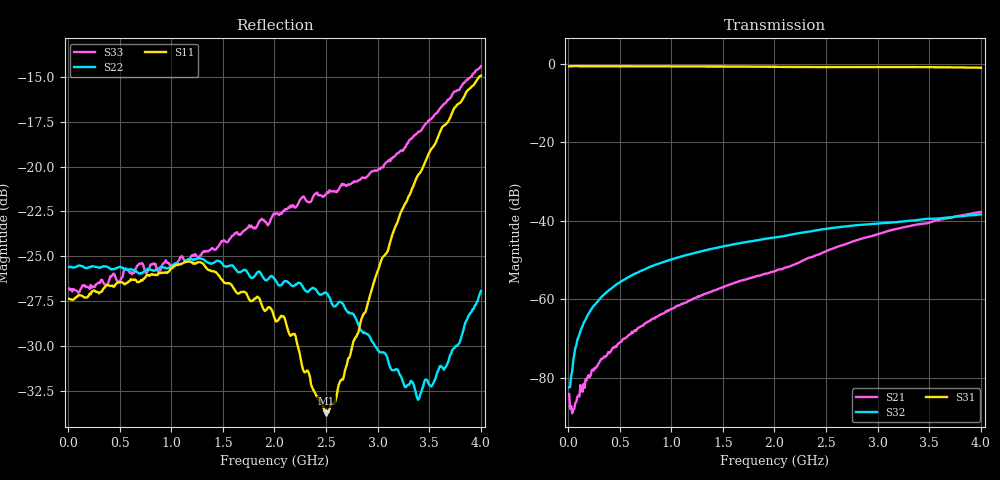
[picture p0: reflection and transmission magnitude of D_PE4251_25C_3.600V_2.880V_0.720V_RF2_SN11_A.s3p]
! Device ID: PE4251_SoldCshunt_081809
! Dir: c:\Test Bench Repositories\Bench_Software_CVI_Version_8\trunk\PSC 4Port_VNA Bench\datalog\4250\TEST\PE4251_SoldCshunt_081809\25C\3p600000\RF2
! Serial: 11
! Insertion: A
! Temp: 25C
! VDD: 3.600
! Control_Hi: 80.000
! Control_Lo: 20.000
! Logic State: RF2
! Port 1: RFC
! Port 2: RF1
! Port 3: RF2
! V1 = 0.72
! V2 = 0.72
! V3 = 0.72
! IDD: 4.934160e-05
! FILE NAME
! DATE 08/18/09  20:13
! CORRECTED  DATA
#  Hz  S  RI  R  50.00
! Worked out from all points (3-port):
!   401 points, 10 MHz to 4 GHz, reference 50 ohm
!   strongest paths, dB at 10 MHz, 1.008 GHz, 2.005 GHz, 3.002 GHz, 4 GHz:
!     S31: -0.6, -0.6, -0.7, -0.8, -0.9
!     S32: -82.5, -49.8, -44.2, -40.7, -38.3
!     S21: -84.2, -62.4, -52.8, -43.4, -37.7
!   lowest |S11| = -33.7 dB at 2.504 GHz (marker M1), VSWR 1.04, Z = 50.5 - j2 ohm
!   |S11| at or under -10 dB: start of sweep to end of sweep
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1e7  0.0428 -0.00063  9.73e-05 6.83e-05  0.9368 -0.00251
     6.12e-05 -8.49e-06  0.0525 -0.000729  3.26e-05 1.67e-05
     0.9381 -0.00458  5.86e-06 -7.49e-05  0.0457 0.000517
8.98e7  0.0435 0.00135  1.78e-05 -5.36e-05  0.9389 -0.0323
        2.09e-05 -5.28e-05  0.0528 -0.00117  3.32e-05 0.000282
        0.939 -0.0326  4.61e-05 0.000301  0.0449 -0.000647
1.696e8  0.0432 0.0021  2.64e-06 -8.73e-05  0.9367 -0.059
         1.02e-05 -9.56e-05  0.0522 -0.000973  5.14e-05 0.000563
         0.937 -0.06  5.4e-05 0.00055  0.0462 0.00115
2.893e8  0.0446 0.0029  -4.11e-05 -0.000147  0.9329 -0.1015
         -4.97e-05 -0.000139  0.0524 -0.00232  7.87e-05 0.000952
         0.9328 -0.1011  7.88e-05 0.000938  0.0473 -0.000288
4.888e8  0.0477 0.00134  -0.000155 -0.000217  0.9205 -0.1684
         -0.000158 -0.000224  0.0523 -0.00485  0.00015 0.00159
         0.921 -0.1675  0.000157 0.0016  0.0473 -0.00441
1.077325e9  0.0522 -0.0112  -0.00077 -0.000323  0.8615 -0.3564
            -0.000769 -0.000333  0.0522 -0.0116  0.000513 0.00342
            0.8631 -0.3557  0.000508 0.00342  0.0541 -0.00981
2.005e9  0.035 -0.0137  -0.00224 -0.000415  0.6957 -0.6032
         -0.00224 -0.000417  0.0479 -0.00694  0.00116 0.00603
         0.6977 -0.6038  0.00117 0.00605  0.0665 -0.0317
2.50375e9  0.00571 -0.0197  -0.00402 -0.000852  0.5859 -0.7012
           -0.00404 -0.000857  0.0444 4.22e-05  0.00158 0.00777
           0.5876 -0.7011  0.00158 0.00777  0.053 -0.0653
3.391525e9  -0.0866 -0.0384  -0.009 0.001  0.3472 -0.8441
            -0.00898 0.000991  0.0131 0.0182  0.00231 0.00999
            0.35 -0.8439  0.00229 0.01  -0.0267 -0.122
4e9  -0.177 -0.0268  -0.0126 0.00363  0.1323 -0.8873
     -0.0125 0.0036  -0.0262 0.0366  0.00243 0.0118
     0.1343 -0.8863  0.00243 0.0118  -0.1336 -0.1355
